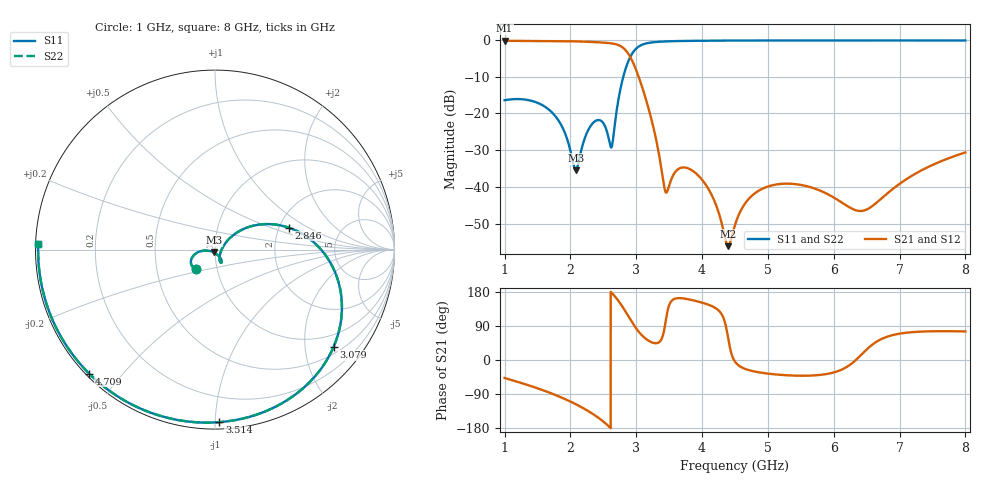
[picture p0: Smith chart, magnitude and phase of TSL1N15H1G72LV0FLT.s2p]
! TSL1N15H1G72LV0FLT  S-PARAMETER MODEL  ( General Type )
! Model Generated by TAIYO YUDEN Corporation (https://www.yuden.co.jp/en/)
! Version 1.0
! TAIYO YUDEN Control No. 160329
! Copyright(c) 2016 TAIYO YUDEN CO.,LTD. All Rights Reserved.
! Products Name : Multilayer Ceramic Devices
! Characteristics :
!  Passband freq : 1426-2200MHz ( At Passband , Insertion Loss : 0.75dB , VSWR 2.0 ),
!  Attenuation : 25dB min at 3400-3800MHz , 25dB min at 4000-5850MHz , Impedance : 50 Ohm ,
!  Case Size : 1.0 x 0.5 / 0.039 x 0.02 [mm/inch] , Thickness : 0.4 / 0.016 [mm/inch]
!  (Conditions: Temperature = 25 degC , DC Bias Current/Voltage = 0A / 0V)
! External Node Assignments :
!  1  o---|-------|---o  2
!  |  LPF  |
! GND o---|-------|---o GND
! Frequency Range : 1GHz  -  8GHz  [ 7001 STEP ]
# MHZ S RI R 50
! Freq[MHz].  S11 Real  S11 Imag  S21 Real  S21 Imag  S12 Real  S12 Imag  S22 Real  S22 Imag
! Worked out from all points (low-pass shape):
!   7001 points, 1 GHz to 8 GHz, reference 50 ohm
!   highest |S21| = -0.21 dB at 1 GHz (marker M1); lowest = -56.1 dB at 4.4 GHz (marker M2)
!   |S21| within 3 dB of the highest: start of sweep to 2.858 GHz
!   lowest |S11| = -35.5 dB at 2.08 GHz (marker M3), VSWR 1.03, Z = 49.2 - j1.49 ohm
!   |S11| at or under -10 dB: start of sweep to 2.803 GHz
!   |S22| runs from -35.1 to -0.1 dB; largest |S21 - S12| = 0
!   S11 on the Smith chart (normalised r, x): 1 GHz: 0.79, -0.18; 2.846 GHz: 2.25, +0.67; 3.079 GHz: 0.66, -2.65; 3.514 GHz: 0.04, -1.03; 4.709 GHz: 0.01, -0.41; 8 GHz: 0.01, +0.02
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1000  -0.1052 -0.109  0.6598 -0.719  0.6598 -0.719  -0.1051 -0.1092
1708  -0.1041 -0.0195  0.035 -0.9658  0.035 -0.9658  -0.1041 -0.0201
2080  -0.00742 -0.0152  -0.4275 -0.8574  -0.4275 -0.8574  -0.00782 -0.0158
2167  0.0144 -0.0289  -0.5393 -0.7861  -0.5393 -0.7861  0.0139 -0.0295
2411  0.0366 -0.0725  -0.8133 -0.4565  -0.8133 -0.4565  0.0359 -0.0729
2624  0.0339 -0.0079  -0.8994 0.0351  -0.8994 0.0351  0.0331 -0.00781
2846  0.4098 0.1226  -0.4107 0.583  -0.4107 0.583  0.4094 0.123
2964  0.6851 -0.1711  -0.0156 0.4638  -0.0156 0.4638  0.6851 -0.1707
3079  0.6607 -0.5423  0.0975 0.2237  0.0975 0.2237  0.6607 -0.5421
3334  0.2641 -0.9078  0.0221 0.0226  0.0221 0.0226  0.2642 -0.9077
3438  0.1187 -0.9489  -0.000431 0.00887  -0.000431 0.00887  0.1189 -0.9488
3514  0.025 -0.9613  -0.0099 0.00565  -0.0099 0.00565  0.0252 -0.9612
3687  -0.1548 -0.9573  -0.0175 0.00536  -0.0175 0.00536  -0.1545 -0.9573
3954  -0.3635 -0.9067  -0.0125 0.00621  -0.0125 0.00621  -0.363 -0.9068
4181  -0.495 -0.8461  -0.00505 0.00432  -0.00505 0.00432  -0.4945 -0.8464
4400  -0.5941 -0.7825  0.000926 0.00126  0.000926 0.00126  -0.5935 -0.7829
4500  -0.6322 -0.7529  0.00302 -0.000226  0.00302 -0.000226  -0.6316 -0.7534
4709  -0.7005 -0.6914  0.00615 -0.00309  0.00615 -0.00309  -0.6999 -0.692
5667  -0.8864 -0.4323  0.0074 -0.00643  0.0074 -0.00643  -0.8858 -0.4335
6392  -0.9498 -0.2659  0.00465 0.000758  0.00465 0.000758  -0.9494 -0.2675
6834  -0.9705 -0.1754  0.00387 0.00751  0.00387 0.00751  -0.9701 -0.1772
8000  -0.9849 0.0311  0.00745 0.0286  0.00745 0.0286  -0.985 0.0289
